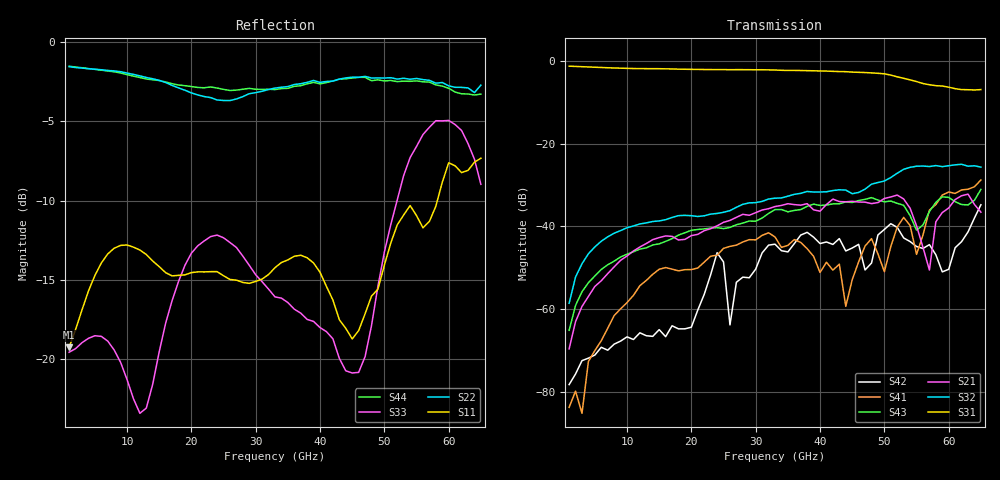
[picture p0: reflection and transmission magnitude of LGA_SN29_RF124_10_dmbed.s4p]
! Created Thu Nov 10 13:45:16 2022
# hz S ma R 50
! 4 Port Network Data from SP1.SP block
! freq  magS11  angS11  magS12  angS12  magS13  angS13  magS14  angS14
!  magS21  angS21  magS22  angS22  magS23  angS23  magS24  angS24
!  magS31  angS31  magS32  angS32  magS33  angS33  magS34  angS34
!  magS41  angS41  magS42  angS42  magS43  angS43  magS44  angS44
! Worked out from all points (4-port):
!   65 points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, 1 GHz to 65 GHz, reference 50 ohm
!   strongest paths, dB at 1 GHz, 17 GHz, 33 GHz, 49 GHz, 65 GHz:
!     S31: -1.3, -2.0, -2.3, -3.0, -7.0
!     S32: -58.6, -37.9, -33.2, -29.4, -25.7
!     S21: -69.6, -42.4, -35.2, -34.3, -36.6
!     S43: -65.1, -43.0, -36.0, -33.7, -31.1
!     S41: -83.7, -50.3, -42.6, -46.7, -28.8
!     S42: -78.2, -64.0, -44.3, -42.1, -34.8
!   lowest |S11| = -19.2 dB at 1 GHz (marker M1), VSWR 1.25, Z = 60.4 - j6.15 ohm
!   |S11| at or under -10 dB: start of sweep to 58.23 GHz
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1e9  0.1092 -27.4  0.0002693 -105.3  0.8598 -13.7  0.000111 6.4
     0.0003315 -100.1  0.836 171.1  0.001219 77.1  0.0001379 84.1
     0.8586 -13.7  0.001176 72.0  0.1053 -26.7  0.0005502 69.7
     6.517e-05 -110.4  0.0001227 102.1  0.0005546 60.5  0.839 171.3
8e9  0.224 -132.0  0.003157 133.7  0.8176 -104.6  0.0008193 105.2
     0.003239 133.5  0.8106 110.4  0.00827 -0.4  0.0004851 0.5
     0.8164 -104.6  0.008256 -0.5  0.1071 -160.8  0.003826 -14.7
     0.0008357 103.4  0.0003778 6.6  0.003799 -14.1  0.8055 112.0
1.9e10  0.1846 169.0  0.00678 -25.8  0.7891 114.7  0.002946 -31.8
        0.006955 -25.7  0.7047 2.8  0.01363 -130.6  0.0005457 -156.8
        0.788 114.9  0.01357 -130.4  0.1978 154.3  0.008421 -151.3
        0.003 -32.8  0.0005786 -149.3  0.008361 -151.1  0.7283 3.0
3.4e10  0.202 -46.0  0.01841 136.3  0.766 -81.4  0.005547 79.5
        0.01788 134.8  0.7201 -172.6  0.02206 61.4  0.00539 -1.1
        0.7656 -81.3  0.02202 61.7  0.1559 14.2  0.01628 28.1
        0.005568 81.6  0.005078 -4.4  0.01593 29.8  0.713 -162.9
4.7e10  0.1392 -147.8  0.01977 -25.9  0.7209 98.4  0.005602 66.0
        0.01958 -27.3  0.7793 71.6  0.02825 -58.2  0.003291 -149.6
        0.7193 98.6  0.02813 -58.5  0.1019 130.8  0.02145 -131.8
        0.005787 67.6  0.002971 -153.0  0.02118 -132.7  0.7737 73.3
5.5e10  0.2838 167.4  0.01087 -173.2  0.5605 -21.3  0.00413 -23.4
        0.01016 -168.0  0.7674 1.5  0.05269 -161.5  0.005622 122.4
        0.5599 -21.0  0.05317 -161.2  0.4687 -55.1  0.008103 117.2
        0.004588 -17.6  0.005706 113.2  0.00898 111.4  0.7541 3.2
6.5e10  0.4302 140.0  0.01339 167.8  0.4484 -154.9  0.03483 -126.3
        0.01483 163.0  0.731 -131.1  0.05083 32.7  0.01653 169.8
        0.4475 -154.3  0.05183 34.1  0.356 -156.1  0.0291 17.7
        0.03625 -123.9  0.01821 169.8  0.02792 16.9  0.685 -126.0
